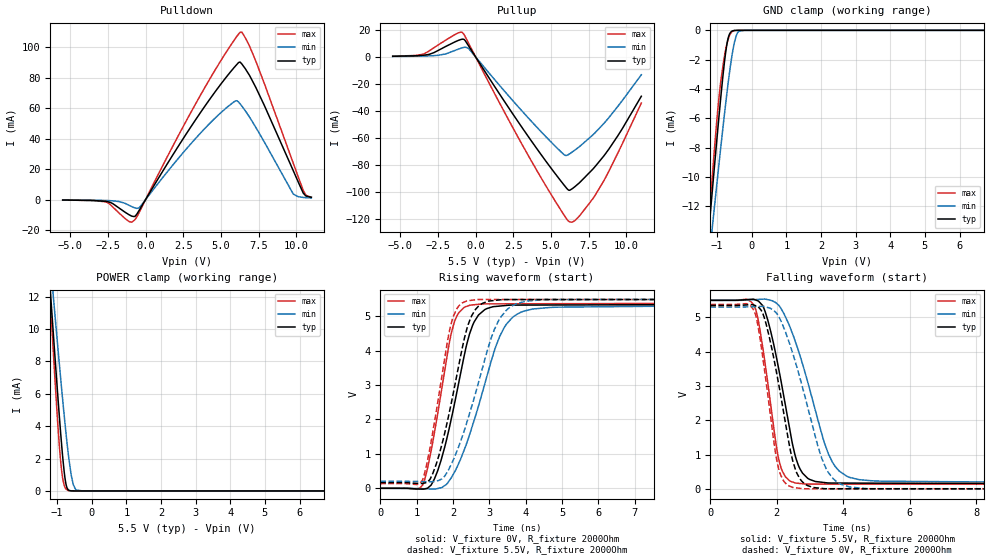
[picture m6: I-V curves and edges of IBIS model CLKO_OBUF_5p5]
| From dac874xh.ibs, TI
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|   CLKO_OBUF_5p5 Model
[Model]   CLKO_OBUF_5p5
Model_type   3-state
Polarity   Non-Inverting
Vmeas = 2.75
Vref = 0
Cref = 2pF
Rref = 100000
|   typ   min   max
C_comp   5.38106E-13   4.41371E-13  5.81321E-13
| Where nom  PVT is Nominal Process, 5.5V, 27C
|   Fast PVT is Strong Process,  5.501V, -40C
|   Slow PVT is Weak Process,   5.499V, 150C
[Voltage Range]   5.5   5.499   5.501
[Temperature Range]   27   150   -40
[Pullup Reference]   5.5   5.499   5.501
[Pulldown Reference]   0   -0   0
[Power Clamp Reference]   5.5   5.499   5.501
[GND Clamp Reference]   0   0   0
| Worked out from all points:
|   slope of the pulldown table from 0 to 0.825 V, typ, clamps not added: 60.9 ohm
|   slope of the pullup table from 0 to 0.825 V, typ, clamps not added: 57.3 ohm
|   GND clamp passes 1 mA (typ) near -0.72 V on its own axis
|   POWER clamp passes 1 mA (typ) near -0.79 V on its own axis
|   falling waveform, V_fixture 5.5V, R_fixture 2000Ohm: 20-80 % time 635ps typ, 956ps min, 465ps max; typ from 5.5 V to 0.161 V
|   rising waveform, V_fixture 0V, R_fixture 2000Ohm: 20-80 % time 663ps typ, 934ps min, 518ps max; typ from 0 V to 5.35 V
|   rising waveform, V_fixture 5.5V, R_fixture 2000Ohm: 20-80 % time 649ps typ, 903ps min, 503ps max; typ from 0.161 V to 5.5 V
|   falling waveform, V_fixture 0V, R_fixture 2000Ohm: 20-80 % time 612ps typ, 914ps min, 449ps max; typ from 5.35 V to 0 V
[Pulldown]
|   Voltage   I(typ)   I(min)   I(max)
-5.5V     -274.3uA   -207.4uA   -262.6uA
-2.646V   -1.15mA    -566.8uA   -1.494mA
-1.144V   -9.64mA    -3.497mA   -14.05mA
-748mV    -11.13mA   -5.296mA   -13.55mA
-368.5mV  -6.102mA   -4.706mA   -7.288mA
4.763V    72.64mA    54.83mA    87.35mA
5.951V    87.41mA    64.59mA    105.5mA
6.38V     89.02mA    61.44mA    109.8mA
7.354V    72.77mA    46.74mA    89.79mA
9.796V    19.1mA     3.78mA     24.04mA
10.47V    4.145mA    1.408mA    5.889mA
11V       1.492mA    1.043mA    1.534mA
[GND Clamp]
|   Voltage   I(typ)   I(min)   I(max)
-5.5V     -135.3mA   -117mA     -157.1mA
-1.375V   -17.34mA   -18.78mA   -17.39mA
-1.21V    -12.8mA    -14.99mA   -12.09mA
-1.127V   -10.56mA   -13.11mA   -9.522mA
-979mV    -6.643mA   -9.78mA    -5.309mA
-880mV    -4.172mA   -7.614mA   -3.19mA
-715mV    -881.2uA   -4.192mA   -881.7uA
-649mV    -281.2uA   -2.954mA   -380.5uA
-550mV    -34.24uA   -1.391mA   -53.46uA
-418mV    -1.221uA   -193.5uA   -1.154uA
-220mV    0A         -1.089uA   0A
11V       0A         0A         0A
[Pullup]
|   Voltage   I(typ)   I(min)   I(max)
-5.5V     439.1uA    307.5uA    504.8uA
-3.454V   1.199mA    611.2uA    2.085mA
-863.5mV  13.15mA    6.807mA    17.92mA
-451mV    7.94mA     6.06mA     9.848mA
2.7V      -46.13mA   -35.38mA   -57.18mA
5.242V    -86.01mA   -65.75mA   -106.3mA
5.934V    -95.98mA   -73mA      -118.4mA
6.248V    -98.95mA   -71.84mA   -122.5mA
6.859V    -93.73mA   -66.9mA    -118.5mA
7.915V    -81.64mA   -56.47mA   -103.1mA
9.432V    -58.68mA   -36.83mA   -71.59mA
11V       -29.22mA   -13.28mA   -34.3mA
[POWER Clamp]
|   Voltage   I(typ)   I(min)   I(max)
-5.5V     153.2mA    129.9mA    181.8mA
-1.21V    12.73mA    14.42mA    12.18mA
-1.161V   11.2mA     13.2mA     10.34mA
-1.095V   9.187mA    11.59mA    7.945mA
-979mV    5.766mA    8.806mA    4.015mA
-896.5mV  3.478mA    6.872mA    1.751mA
-847mV    2.232mA    5.744mA    857.4uA
-781mV    884.2uA    4.295mA    252.8uA
-682mV    66.16uA    2.324mA    28.67uA
-533.5mV  660.3nA    379.7uA    346.6nA
-269.5mV  0A         430.8nA    0A
11V       0A         0A         0A
[Ramp]
R_load = 2000
|   typ   min   max
dV/dt_r   3.2087/6.60245e-10   3.18158/9.28473e-10   3.22672/5.16642e-10
dV/dt_f   3.20332/6.33481e-10   3.17625/9.54121e-10   3.21936/4.63754e-10
[Falling Waveform]
V_fixture = 5.5V
V_fixture_min = 5.499V
V_fixture_max = 5.501V
R_fixture = 2000Ohm
C_fixture = 0F
|   Time   V(typ)   V(min)   V(max)
0s        5.5V       5.499V     5.501V
1.223ns   5.53V      5.515V     5.458V
1.399ns   5.497V     5.524V     5.118V
1.586ns   5.326V     5.534V     4.077V
2.115ns   3.219V     5.282V     665.2mV
2.542ns   1.021V     4.344V     186.4mV
2.873ns   371.3mV    3.318V     148.2mV
3.763ns   178mV      653.1mV    148.1mV
5.163ns   174.5mV    232.6mV    147.9mV
125ns     161.1mV    205.2mV    135.4mV
[Rising Waveform]
V_fixture = 0V
V_fixture_min = 0V
V_fixture_max = 0V
R_fixture = 2000Ohm
C_fixture = 0F
|   Time   V(typ)   V(min)   V(max)
0s        1.894nV    33.27nV    1.743nV
1.09ns    -22.05mV   -8.852mV   6.956mV
1.414ns   119.8mV    -20.86mV   1.17V
1.671ns   806.3mV    15.66mV    2.756V
2.04ns    2.443V     465.9mV    4.833V
2.457ns   4.49V      1.557V     5.319V
2.802ns   5.128V     2.762V     5.359V
3.477ns   5.317V     4.778V     5.363V
4.899ns   5.329V     5.266V     5.366V
125ns     5.348V     5.303V     5.378V
[Rising Waveform]
V_fixture = 5.5V
V_fixture_min = 5.499V
V_fixture_max = 5.501V
R_fixture = 2000Ohm
C_fixture = 0F
|   Time   V(typ)   V(min)   V(max)
0s        161.1mV    205.2mV    135.4mV
1.09ns    140.6mV    197.5mV    146.9mV
1.374ns   271.9mV    190mV      1.21V
1.621ns   982mV      234.4mV    2.764V
1.996ns   2.692V     792.1mV    4.952V
2.382ns   4.633V     1.913V     5.448V
2.678ns   5.266V     2.978V     5.489V
3.317ns   5.481V     4.98V      5.489V
4.57ns    5.487V     5.485V     5.489V
125ns     5.5V       5.499V     5.501V
[Falling Waveform]
|Gnd
V_fixture = 0V
V_fixture_min = 0V
V_fixture_max = 0V
R_fixture = 2000Ohm
C_fixture = 0F
|   Time   V(typ)   V(min)   V(max)
0s        5.348V     5.303V     5.378V
1.21ns    5.374V     5.313V     5.337V
1.38ns    5.339V     5.319V     5.01V
1.553ns   5.173V     5.325V     4.021V
2.073ns   2.972V     5.001V     539.5mV
2.477ns   836.2mV    3.964V     51.7mV
2.802ns   187.3mV    2.862V     10.62mV
3.549ns   12.6mV     488.5mV    10.56mV
4.783ns   12.47mV    12.39mV    10.45mV
125ns     1.901nV    33.25nV    1.745nV
